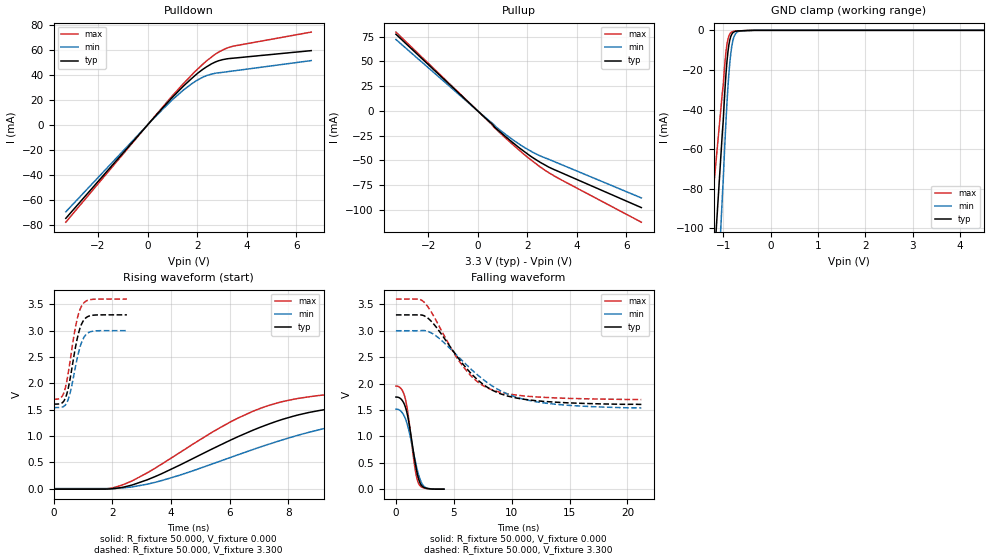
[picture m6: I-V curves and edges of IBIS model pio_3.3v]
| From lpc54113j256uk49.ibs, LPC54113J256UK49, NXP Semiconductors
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[Model]   pio_3.3v
Model_type I/O
Vinl=8.000E-01
Vinh=2.000E+00
Vref=0.000E+00
Rref=1.000E+06
Cref=2.000E-11
Vmeas=1.650E+00
C_comp   9.060E-13   8.700E-13   9.240E-13
[Voltage Range]   3.300E+00   3.000E+00   3.600E+00
[POWER Clamp Reference]   3.300E+00   3.000E+00   3.600E+00
[GND Clamp Reference]   0.000E+00   0.000E+00   0.000E+00
[Pullup Reference]   3.300E+00   3.000E+00   3.600E+00
[Pulldown Reference]   0.000E+00   0.000E+00   0.000E+00
[Temperature Range]   25   105   -40
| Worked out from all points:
|   slope of the pulldown table from 0 to 0.495 V, typ, clamps not added: 44.8 ohm
|   slope of the pullup table from 0 to 0.495 V, typ, clamps not added: 43.6 ohm
|   GND clamp passes 1 mA (typ) near -0.79 V on its own axis
|   rising waveform, R_fixture 50.000, V_fixture 0.000: 20-80 % time 4.35ns typ, 5.29ns min, 3.74ns max; typ from -0.012 V to 1.73 V
|   falling waveform, R_fixture 50.000, V_fixture 0.000: 20-80 % time 788ps typ, 920ps min, 704ps max; typ from 1.74 V to 0 V
|   rising waveform, R_fixture 50.000, V_fixture 3.300: 20-80 % time 341ps typ, 343ps min, 341ps max; typ from 1.6 V to 3.3 V
|   falling waveform, R_fixture 50.000, V_fixture 3.300: 20-80 % time 3.95ns typ, 4.88ns min, 3.41ns max; typ from 3.3 V to 1.6 V
[GND Clamp]
-3.3V     -913.2mA   -1.204A    -624.3mA
-1.02V    -52.03mA   -84.42mA   -31.74mA
-1V       -45.42mA   -75.21mA   -27.57mA
-960mV    -28.37mA   -54.32mA   -15.06mA
-920mV    -15.3mA    -36.02mA   -6.838mA
-880mV    -7.16mA    -21.59mA   -2.755mA
-860mV    -4.693mA   -16.01mA   -1.759mA
-820mV    -1.962mA   -8.078mA   -817.1uA
-780mV    -892.3uA   -3.719mA   -513.8uA
-740mV    -500.1uA   -1.659mA   -382.6uA
-520mV    -119.4uA   -145.6uA   -106.5uA
6.6V      0A         0A         0A
[Power Clamp]
-3.3V     0A         0A         0A
0V        0A         0A         0A
3.3V      0A         0A         0A
6.6V      0A         0A         0A
[Pullup]
-3.3V     77.49mA    72.2mA     79.65mA
760mV     -18.12mA   -16.61mA   -18.86mA
1.46V     -32.91mA   -29.95mA   -34.98mA
2.12V     -45.48mA   -40.34mA   -48.91mA
2.58V     -52.8mA    -46.08mA   -57.61mA
3.14V     -59.87mA   -51.73mA   -66.48mA
6.6V      -97.67mA   -87.89mA   -112.4mA
[Pulldown]
-3.3V     -74.59mA   -69.4mA    -77.67mA
140mV     3.186mA    2.948mA    3.327mA
940mV     20.73mA    18.9mA     21.9mA
1.44V     30.86mA    27.69mA    32.8mA
1.78V     37.07mA    32.83mA    39.81mA
2.24V     44.5mA     38.17mA    48.65mA
2.78V     50.6mA     41.38mA    57.01mA
3.34V     53.01mA    42.75mA    62.23mA
6.6V      59.25mA    51.3mA     74.05mA
[Rising Waveform]
R_fixture = 50.000
V_fixture = 0.000
V_fixture_min = 0.000
V_fixture_max = 0.000
|  time   V(typ)   V(min)   V(max)
0s        -11.6mV    0V         -11.05mV
1.75ns    -10.32mV   -333.1uV   -6.202mV
2.35ns    23.6mV     11.86mV    69.84mV
3.7ns     286.1mV    153.6mV    469.2mV
6.3ns     989.1mV    644.7mV    1.343V
7.3ns     1.218V     836mV      1.572V
8.35ns    1.4V       1.016V     1.713V
10.15ns   1.565V     1.242V     1.825V
12.3ns    1.648V     1.381V     1.882V
20.7ns    1.733V     1.516V     1.939V
[Falling Waveform]
R_fixture = 50.000
V_fixture = 0.000
V_fixture_min = 0.000
V_fixture_max = 0.000
|  time   V(typ)   V(min)   V(max)
0s        1.744V     1.516V     1.952V
450ps     1.704V     1.472V     1.902V
800ps     1.565V     1.346V     1.721V
1.1ns     1.286V     1.129V     1.338V
1.65ns    518.3mV    554.8mV    392mV
1.8ns     338.9mV    407.2mV    218.3mV
1.95ns    201.2mV    279.8mV    112.6mV
2.2ns     74.53mV    126.4mV    42.69mV
2.55ns    23.21mV    31.51mV    15.22mV
4.15ns    0V         0V         0V
[Rising Waveform]
R_fixture = 50.000
V_fixture = 3.300
V_fixture_min = 3.000
V_fixture_max = 3.600
|  time   V(typ)   V(min)   V(max)
0s        1.605V     1.538V     1.697V
250ps     1.615V     1.542V     1.724V
400ps     1.711V     1.584V     1.907V
550ps     2.039V     1.781V     2.367V
750ps     2.691V     2.319V     3.076V
850ps     2.949V     2.579V     3.315V
1ns       3.174V     2.835V     3.506V
1.15ns    3.262V     2.948V     3.573V
1.3ns     3.29V      2.985V     3.593V
2.5ns     3.3V       3V         3.6V
[Falling Waveform]
R_fixture = 50.000
V_fixture = 3.300
V_fixture_min = 3.000
V_fixture_max = 3.600
|  time   V(typ)   V(min)   V(max)
0s        3.3V       3V         3.6V
2.4ns     3.287V     3.004V     3.548V
3.45ns    3.078V     2.905V     3.202V
4.85ns    2.646V     2.628V     2.635V
5.8ns     2.365V     2.418V     2.323V
6.9ns     2.102V     2.191V     2.059V
8.15ns    1.896V     1.979V     1.894V
9.75ns    1.758V     1.791V     1.802V
12.1ns    1.675V     1.655V     1.747V
21.2ns    1.605V     1.538V     1.697V
[Ramp]
dV/dt_r   1.0470E+00/4.3389E-09   9.0819E-01/5.2888E-09   1.1703E+00/3.7398E-09
dV/dt_f   1.0173E+00/3.9512E-09   8.7689E-01/4.8527E-09   1.1419E+00/3.3989E-09
R_load = 50
